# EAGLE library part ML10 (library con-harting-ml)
HARTING
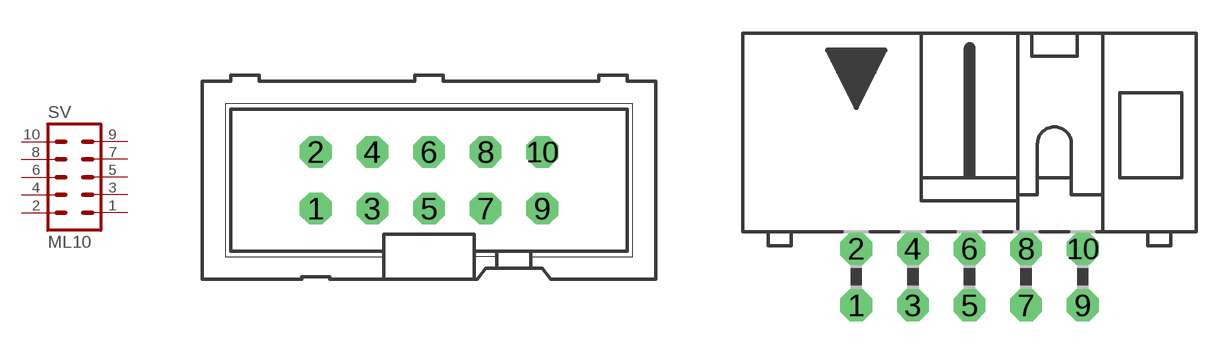
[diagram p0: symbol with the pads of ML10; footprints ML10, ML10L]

Designator prefix SV

## ML10 (OC_FARNELL: unknown; OC_NEWARK: unknown)  [ML10]
1  1  pas
2  2  pas
3  3  pas
4  4  pas
5  5  pas
6  6  pas
7  7  pas
8  8  pas
9  9  pas
10  10  pas

## ML10L (OC_FARNELL: unknown; OC_NEWARK: unknown)  [ML10L]
Pads as for ML10

## ML10-3M (OC_FARNELL: unknown; OC_NEWARK: unknown)  [3M_10]
Pads as for ML10

## ML10-3ML (OC_FARNELL: unknown; OC_NEWARK: unknown)  [3M_10L]
Pads as for ML10

## Footprint ML10 (pad centres in mm)
HARTING
drill 0.914 octagon: 1 -5.08,-1.27; 2 -5.08,1.27; 3 -2.54,-1.27; 4 -2.54,1.27; 5 0,-1.27; 6 0,1.27; 7 2.54,-1.27; 8 2.54,1.27; 9 5.08,-1.27; 10 5.08,1.27

## Footprint ML10L (pad centres in mm)
HARTING
drill 0.914 octagon: 1 -5.08,-1.27; 2 -5.08,1.27; 3 -2.54,-1.27; 4 -2.54,1.27; 5 0,-1.27; 6 0,1.27; 7 2.54,-1.27; 8 2.54,1.27; 9 5.08,-1.27; 10 5.08,1.27

## Footprint 3M_10 (pad centres in mm)
3M
drill 0.813 square: 1 -5.08,-1.27; 2 -5.08,1.27; 3 -2.54,-1.27; 4 -2.54,1.27; 5 0,-1.27; 6 0,1.27; 7 2.54,-1.27; 8 2.54,1.27; 9 5.08,-1.27; 10 5.08,1.27

## Footprint 3M_10L (pad centres in mm)
3M
drill 0.813 square: 1 -5.08,-5.08; 2 -5.08,-2.54; 3 -2.54,-5.08; 4 -2.54,-2.54; 5 0,-5.08; 6 0,-2.54; 7 2.54,-5.08; 8 2.54,-2.54; 9 5.08,-5.08; 10 5.08,-2.54
hole 2.54 at -10.998,-3.277
hole 2.54 at 10.998,-3.277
